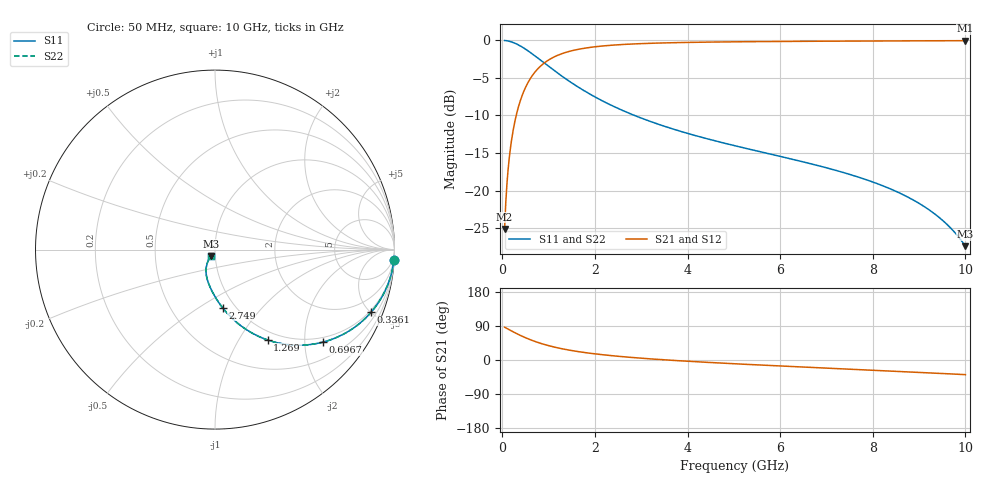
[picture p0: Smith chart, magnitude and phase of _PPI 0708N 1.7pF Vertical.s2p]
! S-Parameter data specifications (vertical orientation):
! Substrate: 40-mil Rogers 3003C, Substrate thickness, H=1.016mm, Dielectric constant, Er=3, Conductor thickness, T_mtl=0.043mm, Loss Tangent, Tand=0.003
! PCB Mounting Pad Footprint: Pad width, PadW=2.54mm , Pad length, PadL=0.51mm , Pad gap, PadG (edge-to-edge)=0.71mm , Reference planes=1.73mm apart
! Created Tue Jan 16 08:43:46 2018
# GHz S MA R 50
! 2 Port Network Data from SP1.SP block
! freq  magS11  angS11  magS21  angS21  magS12  angS12  magS22  angS22
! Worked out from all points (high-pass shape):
!   801 points, 50 MHz to 10 GHz, reference 50 ohm
!   highest |S21| = -0.05 dB at 10 GHz (marker M1); lowest = -25.1 dB at 50 MHz (marker M2)
!   |S21| within 3 dB of the highest: 899.5 MHz to end of sweep
!   lowest |S11| = -27.4 dB at 10 GHz (marker M3), VSWR 1.09, Z = 47.6 - j3.4 ohm
!   |S11| at or under -10 dB: 2.857 GHz to end of sweep
!   |S22| runs from -27.4 to 0.0 dB; largest |S21 - S12| = 0
!   S11 on the Smith chart (normalised r, x): 50 MHz: 1, -34; 336.1 MHz: 0.88, -5.02; 696.8 MHz: 0.88, -2.42; 1.269 GHz: 0.88, -1.34; 2.749 GHz: 0.87, -0.63; 10 GHz: 0.95, -0.07
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0.05  0.9985 -3.4  0.05546 86.6  0.05546 86.6  0.9985 -3.4
0.074875  0.9966 -5.1  0.0829 84.9  0.0829 84.9  0.9966 -5.1
0.124625  0.9905 -8.4  0.1371 81.6  0.1371 81.6  0.9905 -8.4
0.174375  0.9817 -11.7  0.1901 78.3  0.1901 78.3  0.9817 -11.7
0.249  0.9638 -16.5  0.2665 73.5  0.2665 73.5  0.9638 -16.5
0.3360625  0.9369 -21.9  0.3495 68.1  0.3495 68.1  0.9369 -21.9
0.49775  0.8754 -31.1  0.4831 58.9  0.4831 58.9  0.8754 -31.1
0.69675  0.7917 -40.6  0.6104 49.3  0.6104 49.3  0.7917 -40.6
0.9828125  0.6779 -51.5  0.7345 38.4  0.7345 38.4  0.6779 -51.5
1.268875  0.5832 -59.8  0.8116 30.2  0.8116 30.2  0.5832 -59.8
1.716625  0.4724 -69.1  0.8804 20.8  0.8804 20.8  0.4724 -69.1
2.176813  0.3935 -76.1  0.9182 13.8  0.9182 13.8  0.3935 -76.1
2.748937  0.3263 -82.6  0.9439 7.2  0.9439 7.2  0.3263 -82.6
3.370812  0.2764 -88.2  0.9595 1.5  0.9595 1.5  0.2764 -88.2
5.025  0.1988 -99.5  0.9781 -10.0  0.9781 -10.0  0.1988 -99.5
6.691625  0.1501 -108.8  0.9862 -19.6  0.9862 -19.6  0.1501 -108.8
7.624437  0.1248 -113.7  0.9893 -24.8  0.9893 -24.8  0.1248 -113.7
8.345812  0.1037 -117.3  0.9914 -28.9  0.9914 -28.9  0.1037 -117.3
8.868187  0.0868 -119.8  0.9927 -31.8  0.9927 -31.8  0.0868 -119.8
9.3035  0.07124 -121.7  0.9937 -34.4  0.9937 -34.4  0.07124 -121.7
9.65175  0.05759 -122.8  0.9943 -36.5  0.9943 -36.5  0.05759 -122.8
10  0.04268 -123.3  0.9948 -38.7  0.9948 -38.7  0.04268 -123.3
